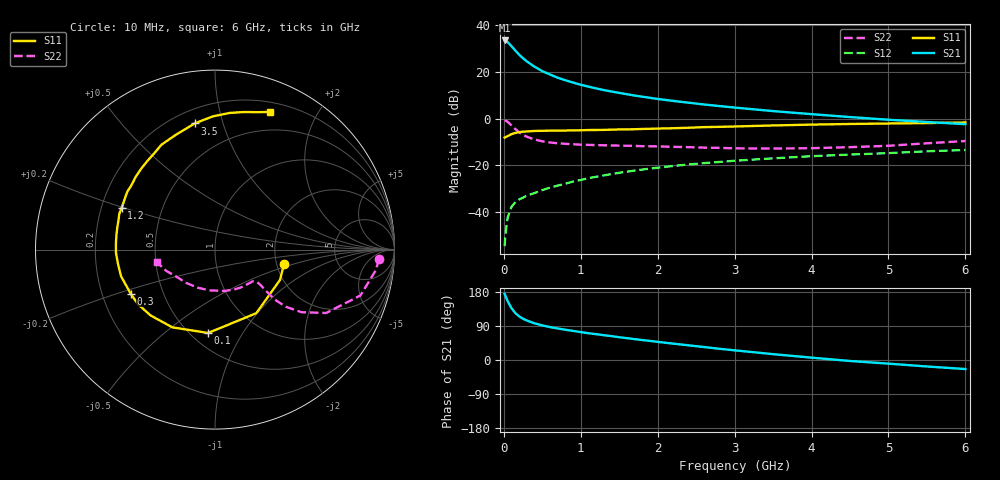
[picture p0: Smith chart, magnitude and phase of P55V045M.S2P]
! SIEMENS Small Signal Semiconductors
! BFP183
! Si NPN RF Bipolar Junction Transistor in SOT143
! VCE = 5 V  IC = 45 mA
! Common Emitter S-Parameters:  March  1996
# GHz  S  MA  R  50
!  f  S11  S21  S12  S22
! GHz  MAG  ANG  MAG  ANG  MAG  ANG  MAG  ANG
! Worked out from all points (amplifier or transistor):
!   36 points, 10 MHz to 6 GHz, reference 50 ohm
!   highest |S21| = 33.3 dB at 10 MHz (marker M1)
!   |S21| within 3 dB of that: start of sweep to 114.3 MHz
!   unconditionally stable (mu >= 1): 502.5 MHz to 5.822 GHz
!   at 250 MHz: K = 0.70, MSG = 29.7 dB, |S12| = -33.7 dB
!   at 1.4 GHz: K = 1.22, MAG = 14.7 dB, |S12| = -23.7 dB
!   at 6 GHz: K = 0.97, MSG = 5.5 dB, |S12| = -13.4 dB
!   S11 on the Smith chart (normalised r, x): 10 MHz: 2.19, -0.42; 100 MHz: 0.61, -0.72; 300 MHz: 0.32, -0.22; 1.2 GHz: 0.29, +0.20; 3.5 GHz: 0.28, +0.81; 6 GHz: 0.30, +1.43
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0.01  0.393 -11.9  46.22 174.6  0.0019 79.8  0.914 -3.2
0.02  0.3997 -25.0  45.99 169.8  0.0033 78.0  0.9047 -7.1
0.05  0.4225 -57.0  42.8 155.2  0.0078 75.0  0.8498 -17.5
0.1  0.466 -94.7  34.8 136.5  0.0131 59.4  0.7129 -29.7
0.15  0.494 -118.7  28.06 123.7  0.0166 53.8  0.595 -35.9
0.2  0.5132 -134.4  22.97 115.0  0.0189 51.5  0.5093 -38.8
0.25  0.5262 -144.7  19.23 108.7  0.0206 51.9  0.4505 -39.7
0.3  0.5299 -152.5  16.47 104.1  0.0229 52.9  0.4087 -39.6
0.4  0.5443 -164.2  12.71 96.7  0.0258 54.2  0.3571 -38.8
0.5  0.5467 -172.1  10.25 91.3  0.0298 55.3  0.3272 -38.0
0.6  0.5521 -178.3  8.684 86.9  0.0337 57.4  0.3088 -37.7
0.7  0.5531 176.2  7.417 83.2  0.0372 57.9  0.297 -37.7
0.8  0.5554 171.5  6.556 79.8  0.0408 59.1  0.2891 -37.9
1.1  0.5692 159.5  4.794 70.6  0.0535 59.2  0.2741 -40.5
1.2  0.5698 156.0  4.387 68.2  0.0574 59.0  0.2715 -41.8
1.7  0.5918 140.3  3.091 55.1  0.0779 56.5  0.2606 -50.5
2.2  0.6214 127.2  2.377 43.2  0.0973 52.4  0.2491 -61.1
2.8  0.6648 112.7  1.848 29.6  0.1186 46.4  0.2367 -76.9
3.5  0.7121 99.1  1.441 15.4  0.1417 40.0  0.2291 -97.9
4.5  0.7659 83.8  1.075 -2.6  0.1705 30.3  0.2454 -131.0
5.5  0.8002 73.1  0.844 -17.1  0.2005 22.1  0.2971 -156.7
6  0.825 68.4  0.758 -23.9  0.2131 17.3  0.3314 -167.7
